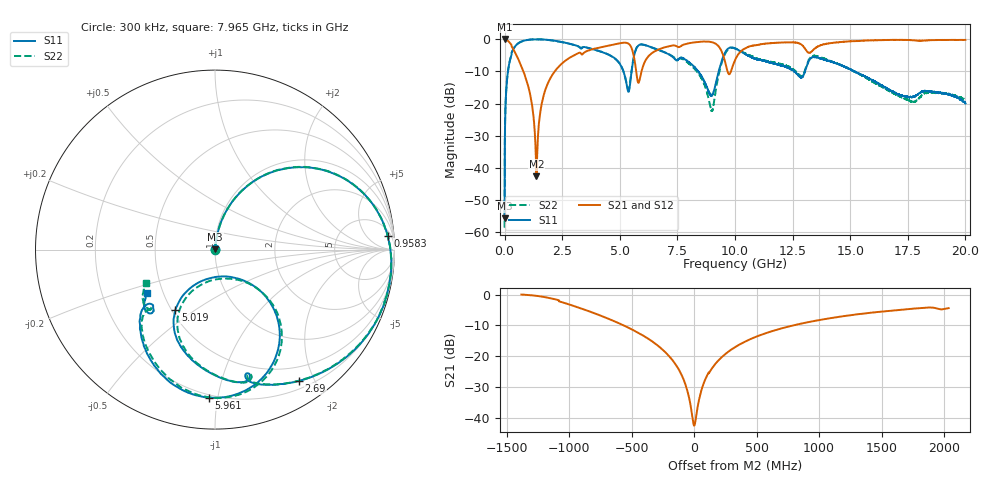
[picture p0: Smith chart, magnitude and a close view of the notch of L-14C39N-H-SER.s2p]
!{L-14C39N}
!Johanson Technology Inc.
!www.johansontechnology.com
!Test Board Conditions:
!Substrate Type  RO4350B
!Substrate Thickness  20 mil
!Substrate Dk  3.66
!TL Type: GCPW
!TL Trace Width  36 mil
!TL Gap  12 mil
!Electrode orientation  Horizontal
!DUT TOPOLOGY	SERIES
!Mounting Pad LxW  26x36 mil
! Created Sun Jun 20 13:05:18 2021
# hz S ma R 50
! 2 Port Network Data from SP1.SP block
! freq  magS11  angS11  magS21  angS21  magS12  angS12  magS22  angS22
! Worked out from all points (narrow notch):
!   20001 points, 300 kHz to 20 GHz, reference 50 ohm
!   highest |S21| = 0.00 dB at 1.3 MHz (marker M1); lowest = -42.6 dB at 1.382 GHz (marker M2)
!   notch at M2: 41.0 dB deep, 339 MHz wide at half that depth
!   lowest |S11| = -55.6 dB at 300 kHz (marker M3), VSWR 1.00, Z = 50.1 + j0.0964 ohm
!   |S11| at or under -10 dB: 8.401 GHz to 9.293 GHz (891.9 MHz wide, 10.1 % of centre); 12.57 GHz to 13.04 GHz (474.7 MHz wide, 3.71 % of centre); 15.17 GHz to end of sweep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
!   |S22| runs from -58.5 to -0.1 dB; largest |S21 - S12| = 0.014
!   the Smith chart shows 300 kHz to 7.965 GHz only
!   S11 on the Smith chart (normalised r, x): 300 kHz: 1.00, +0.00; 958.3 MHz: 10, +21; 2.69 GHz: 0.30, -1.79; 5.019 GHz: 0.52, -0.42; 5.961 GHz: 0.18, -0.94; 7.965 GHz: 0.41, -0.25
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300000  0.001661 35.4  0.9993 -0.1  0.9979 -0.1  0.001187 25.3
1300000  0.002789 91.9  1 -0.2  0.9996 -0.2  0.002907 88.8
1.053e8  0.2345 73.1  0.9619 -14.6  0.9627 -14.5  0.2355 73.1
2.083e8  0.4292 61.1  0.8905 -27.4  0.8913 -27.3  0.4303 61.0
9.583e8  0.965 4.5  0.2248 -83.2  0.2251 -83.4  0.9657 4.5
1.3823e9  0.9901 -13.0  0.007443 -16.2  0.007546 -15.6  0.9899 -12.9
1.7893e9  0.9785 -26.9  0.1713 60.7  0.1718 60.8  0.976 -26.8
2.6903e9  0.8683 -57.4  0.4776 31.4  0.4773 31.3  0.8679 -57.3
3.3343e9  0.7122 -75.1  0.5852 6.9  0.5865 7.0  0.7221 -74.2
5.0193e9  0.4041 -123.2  0.8624 -39.2  0.8638 -39.1  0.4036 -119.9
5.3773e9  0.1517 -84.7  0.8492 -64.1  0.8484 -64.1  0.1652 -81.6
5.6513e9  0.6108 -53.8  0.4465 -93.3  0.447 -93.4  0.6198 -53.1
5.9613e9  0.8247 -92.3  0.3342 -23.4  0.3353 -23.4  0.826 -90.5
6.6673e9  0.6827 -124.2  0.6857 -37.7  0.6872 -37.5  0.6792 -123.0
7.9653e9  0.4485 -147.1  0.8559 -65.9  0.8599 -65.8  0.4263 -154.0
8.9903e9  0.1329 -111.0  0.8971 -101.2  0.8979 -101.3  0.07714 -121.5
9.4313e9  0.4685 -80.9  0.6326 -127.5  0.6356 -127.3  0.4377 -79.9
1.00003e10  0.7182 -139.1  0.4727 -73.8  0.4743 -73.7  0.7164 -143.2
1.12353e10  0.4616 173.2  0.8443 -103.8  0.8472 -104.2  0.4717 168.4
1.33343e10  0.5177 163.5  0.6445 -130.8  0.6426 -131.1  0.5391 165.5
1.66673e10  0.1649 98.0  0.968 176.7  0.9714 177.1  0.1618 81.1
2e10  0.1001 34.8  0.971 126.5  0.9681 126.5  0.1133 52.7
